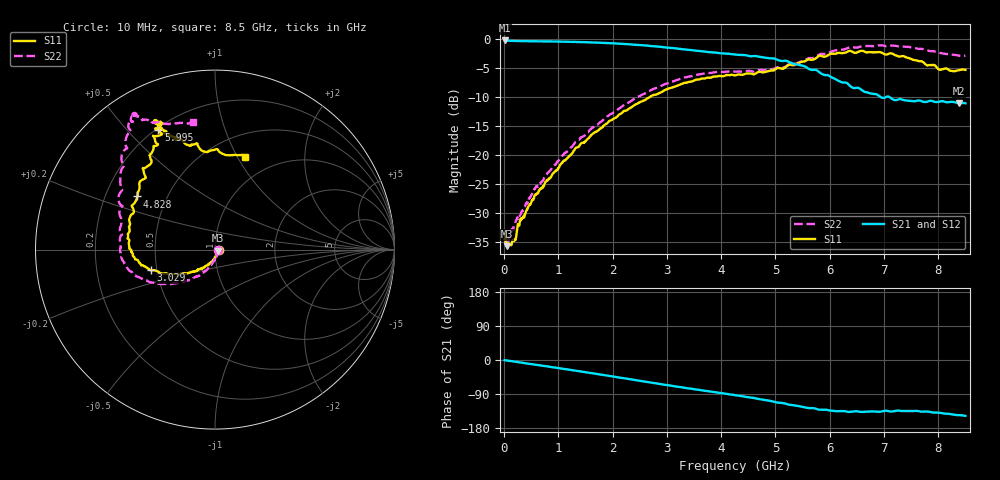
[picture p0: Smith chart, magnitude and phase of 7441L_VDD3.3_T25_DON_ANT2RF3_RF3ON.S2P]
!Agilent Technologies,E5071C,MY46417908,A.11.23
!Date: Mon May 03 19:54:27 2021
!Data & Calibration Information:
!Freq	S11:SOLT2(ON)	S21:SOLT2(ON)	S12:SOLT2(ON)	S22:SOLT2(ON)
!PortZ  Port1:50+j0  Port2:50+j0
!Above PortZ is port z conversion or system Z0 setting when saving the data.
!When reading, reference impedance value at option line is always used.
# Hz S dB R 50
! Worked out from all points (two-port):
!   1601 points, 10 MHz to 8.5 GHz, reference 50 ohm
!   highest |S21| = -0.21 dB at 10 MHz (marker M1); lowest = -11.1 dB at 8.389 GHz (marker M2)
!   |S21| within 3 dB of the highest: start of sweep to 4.815 GHz
!   lowest |S11| = -35.7 dB at 52.45 MHz (marker M3), VSWR 1.03, Z = 51.6 - j0.562 ohm
!   |S11| at or under -10 dB: start of sweep to 2.682 GHz
!   |S22| runs from -35.2 to -1.1 dB; largest |S21 - S12| = 0.003
!   S11 on the Smith chart (normalised r, x): 10 MHz: 1.04, -0.00; 3.029 GHz: 0.46, -0.12; 4.828 GHz: 0.34, +0.28; 5.995 GHz: 0.21, +0.61; 8.5 GHz: 0.73, +1.08
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1e7  -33.60 -1.2  -0.21 -0.4  -0.21 -0.4  -34.74 -10.9
5.245e7  -35.71 -19.4  -0.26 -1.3  -0.27 -1.3  -34.59 -23.0
1.798e8  -34.84 -50.0  -0.29 -4.0  -0.30 -4.0  -32.10 -47.3
2.912312e8  -31.44 -69.3  -0.30 -6.4  -0.31 -6.4  -30.50 -66.5
5.671562e8  -26.91 -89.2  -0.35 -12.1  -0.35 -12.1  -25.71 -88.6
1.087169e9  -21.07 -113.2  -0.42 -23.2  -0.42 -23.2  -19.98 -107.0
1.426769e9  -17.91 -123.7  -0.50 -30.6  -0.50 -30.6  -16.89 -117.6
2.1325e9  -12.92 -143.2  -0.78 -46.5  -0.78 -46.5  -11.87 -134.8
2.843538e9  -9.38 -158.8  -1.28 -62.7  -1.28 -62.8  -8.26 -151.5
3.029256e9  -8.53 -162.2  -1.45 -66.7  -1.45 -66.8  -7.56 -155.7
3.639475e9  -6.79 -175.3  -2.08 -79.9  -2.07 -79.9  -5.98 -168.7
4.255e9  -6.24 167.6  -2.63 -92.8  -2.62 -92.8  -5.60 178.8
4.828075e9  -5.60 145.7  -3.22 -106.1  -3.20 -106.3  -5.33 164.5
5.247269e9  -4.41 131.8  -3.91 -117.8  -3.90 -117.8  -4.34 152.5
5.671769e9  -3.56 118.9  -5.30 -126.8  -5.27 -126.8  -3.25 137.4
5.99545e9  -2.63 115.3  -6.33 -133.1  -6.34 -133.0  -2.28 130.5
6.409338e9  -2.11 115.2  -8.29 -136.3  -8.30 -136.1  -1.36 123.4
7.088538e9  -2.50 114.5  -9.90 -135.2  -9.91 -135.3  -1.15 121.2
7.645694e9  -3.79 109.1  -10.57 -135.3  -10.58 -135.3  -1.65 119.2
8.027744e9  -5.27 95.1  -10.76 -139.2  -10.76 -139.2  -2.33 113.0
8.388569e9  -5.33 76.5  -11.08 -145.4  -11.11 -145.6  -2.85 102.9
8.5e9  -5.28 71.9  -11.05 -147.5  -11.09 -147.7  -2.81 99.8
